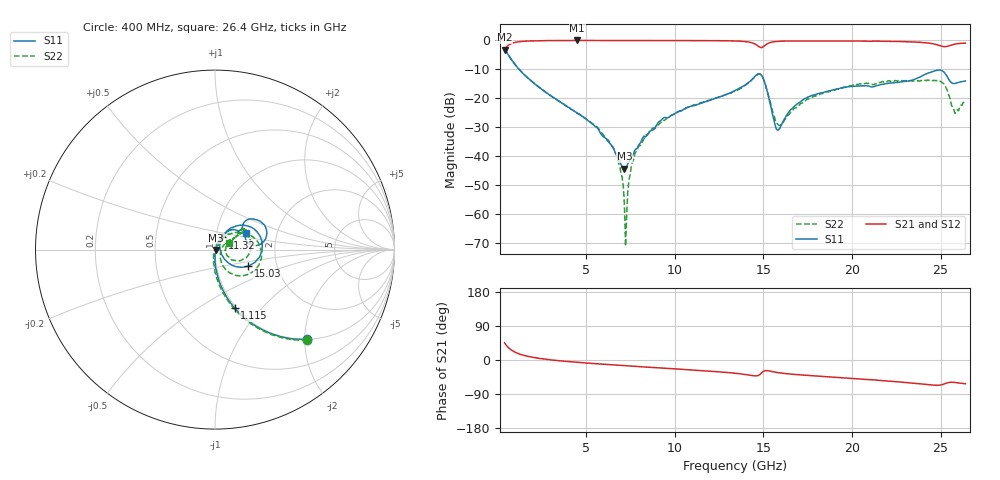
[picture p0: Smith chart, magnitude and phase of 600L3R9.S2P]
!  American Technical Ceramics  Date:  10/27/06
!  One Norden Lane
!  Huntington Station,  NY.  11746-2102
!  Tel:  (631) 622-4700  Fax:  (631) 622-4748
!  Part Number  600L3R9		Mounting Orientation: Vertical
!  Description: Ultra Low ESR Microwave capacitors
!  Application: Coupling, Bypass, Tuning, DC Block
!  Filters, Matching
# GHZ S DB R 50
! Freq  |S11|  S11 Ph  |S21|  S21 Ph  |S12|  S12 Ph  |S22|  S22 Ph
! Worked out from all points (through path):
!   401 points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, 400 MHz to 26.4 GHz, reference 50 ohm
!   highest |S21| = -0.04 dB at 4.495 GHz (marker M1); lowest = -3.2 dB at 400 MHz (marker M2)
!   group delay of S21, straight-line fit = 8.32 ps
!   lowest |S11| = -44.2 dB at 7.16 GHz (marker M3), VSWR 1.01, Z = 50.6 - j0.133 ohm
!   |S11| at or under -10 dB: 1.215 GHz to end of sweep
!   |S22| runs from -71.0 to -2.8 dB; largest |S21 - S12| = 0.0089
!   S11 on the Smith chart (normalised r, x): 400 MHz: 1.00, -2.04; 1.115 GHz: 0.98, -0.72; 11.32 GHz: 1.07, +0.15; 15.03 GHz: 1.43, -0.27; 26.4 GHz: 1.39, +0.27
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0.4  -2.91 -44.4  -3.22 45.0  -3.19 45.0  -2.84 -44.5
1.115  -9.30 -71.5  -0.57 18.0  -0.54 17.9  -9.25 -72.1
4.495  -25.15 -89.7  -0.04 -6.1  -0.02 -6.3  -25.08 -97.1
4.755  -26.09 -90.2  -0.05 -7.1  -0.03 -7.4  -25.97 -99.6
6.575  -37.75 -70.3  -0.04 -13.1  -0.05 -13.5  -37.60 -106.9
6.965  -42.74 -39.2  -0.05 -14.3  -0.06 -14.7  -45.79 -105.5
7.16  -44.22 -12.3  -0.05 -14.9  -0.06 -15.3  -56.66 -72.1
7.29  -43.52 4.6  -0.05 -15.3  -0.06 -15.7  -59.79 60.5
7.485  -41.46 32.7  -0.05 -15.9  -0.07 -16.3  -46.28 51.0
7.875  -37.32 52.6  -0.04 -17.1  -0.07 -17.5  -37.87 55.1
9.11  -28.02 71.0  -0.07 -20.8  -0.10 -21.2  -28.97 52.6
11.32  -22.04 59.0  -0.09 -27.1  -0.11 -27.3  -21.83 54.6
13.4  -17.33 55.7  -0.22 -34.9  -0.24 -35.0  -17.56 43.0
14.7  -11.58 15.2  -1.96 -41.1  -1.99 -41.1  -11.67 -3.3
15.025  -13.64 -26.3  -2.08 -29.5  -2.12 -29.5  -13.62 -45.2
15.805  -31.00 5.7  -0.35 -33.1  -0.39 -33.1  -28.86 -29.7
16.65  -23.30 61.5  -0.22 -37.6  -0.26 -37.5  -24.17 29.9
17.755  -18.99 57.9  -0.19 -41.5  -0.24 -41.4  -19.68 31.6
22.11  -14.76 37.5  -0.36 -55.7  -0.39 -55.5  -13.94 35.7
24.905  -10.23 23.8  -1.71 -66.6  -1.74 -66.1  -14.10 -0.1
25.75  -14.86 18.6  -1.37 -59.0  -1.40 -58.5  -23.97 -9.9
26.4  -14.04 28.1  -0.98 -62.7  -1.00 -62.3  -21.49 26.5
